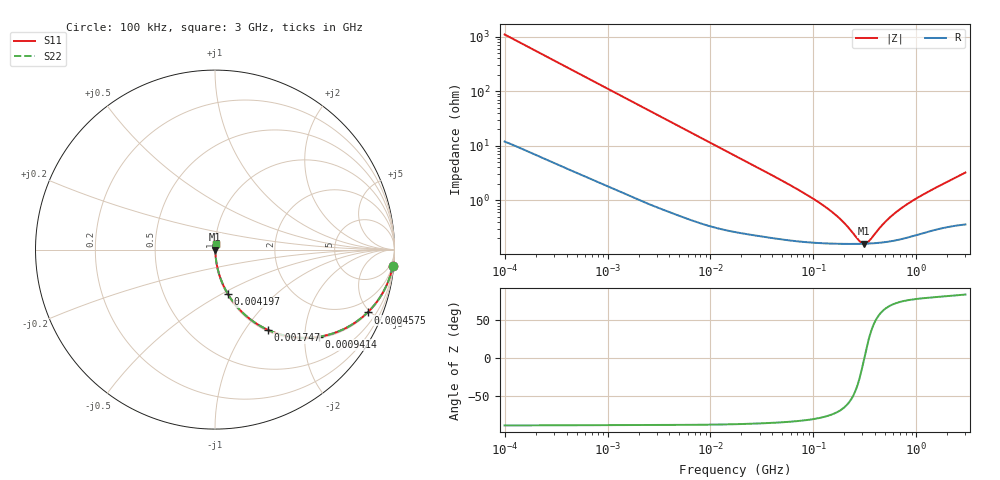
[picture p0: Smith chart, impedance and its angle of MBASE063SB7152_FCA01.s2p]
! MBASE063SB7152_FCA01  S-PARAMETER MODEL  ( Standard Model )
! Model Generated by TAIYO YUDEN Corporation (http://www.ty-top.com)
! Version 1.0
! TAIYO YUDEN Control No. 220601
! Copyright(c) 2020 TAIYO YUDEN CO.,LTD. All Rights Reserved.
! Product Description (link to TY-COMPAS)
! https://ds.yuden.co.jp/TYCOMPAS/or/detail?pn=MBASE063SB7152KFCA01&u=M
! Products Name : Multilayer Ceramic Capacitors
! Characteristics :
!  Capacitance : 1500 [pF] , Rated Voltage : 16 [V] , TCC : X7R
!  Case Size : 0.6 x 0.3 / 0.024 x 0.012 [mm/inch] , Thickness : 0.3 / 0.012 [mm/inch]
!  (Conditions: Temperature = 25 [degC] , DC Bias Voltage = 0 [V])
! External Node Assignments :
!  1  o---| |---o  2
! GND o---------o GND
! Frequency Range : 100kHz  -  3GHz  [ 401 STEP ]
# MHZ S RI R 50
! Freq[MHz].  S11 Real  S11 Imag  S21 Real  S21 Imag  S12 Real  S12 Imag  S22 Real  S22 Imag
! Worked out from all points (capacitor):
!   401 points, 100 kHz to 3 GHz, reference 50 ohm
!   read as one part in series: C = 1.46 nF near 105.3 kHz
!   lowest |Z| = 160 mohm at 310.6 MHz (marker M1)
!   series resonance near 313 MHz, so ESL is about 180 pH
!   S11 on the Smith chart (normalised r, x): 100 kHz: 1, -22; 457.5 kHz: 1.07, -4.83; 941.4 kHz: 1.04, -2.36; 1.747 MHz: 1.02, -1.28; 4.197 MHz: 1.01, -0.54; 3 GHz: 1.01, +0.06
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0.1  0.9907 -0.0907  0.00931 0.0907  0.00931 0.0907  0.9907 -0.0907
0.246461  0.9496 -0.2124  0.0504 0.2124  0.0504 0.2124  0.9496 -0.2124
0.457483  0.85 -0.35  0.15 0.35  0.15 0.35  0.85 -0.35
0.562235  0.7913 -0.3991  0.2087 0.3991  0.2087 0.3991  0.7913 -0.3991
0.941399  0.5812 -0.4854  0.4188 0.4854  0.4188 0.4854  0.5812 -0.4854
1.282589  0.4317 -0.4869  0.5683 0.4869  0.5683 0.4869  0.4317 -0.4869
1.747435  0.2941 -0.4468  0.7059 0.4468  0.7059 0.4468  0.2941 -0.4468
3.161081  0.1174 -0.312  0.8826 0.312  0.8826 0.312  0.1174 -0.312
4.197169  0.0721 -0.2481  0.9279 0.2481  0.9279 0.2481  0.0721 -0.2481
8.202936  0.0223 -0.1349  0.9777 0.1349  0.9777 0.1349  0.0223 -0.1349
17.7727  0.00666 -0.0636  0.9933 0.0636  0.9933 0.0636  0.00666 -0.0636
97.38194  0.00179 -0.0108  0.9982 0.0108  0.9982 0.0108  0.00179 -0.0108
167.3121  0.00162 -0.00499  0.9984 0.00499  0.9984 0.00499  0.00162 -0.00499
210.9903  0.00159 -0.00303  0.9984 0.00303  0.9984 0.00303  0.00159 -0.00303
280.1453  0.00159 -0.000832  0.9984 0.000832  0.9984 0.000832  0.00159 -0.000832
310.5665  0.0016 -5.72e-05  0.9984 5.72e-05  0.9984 5.72e-05  0.0016 -5.72e-05
353.2796  0.00161 0.000912  0.9984 -0.000912  0.9984 -0.000912  0.00161 0.000912
457.1373  0.00168 0.00291  0.9983 -0.00291  0.9983 -0.00291  0.00168 0.00291
547.5153  0.00177 0.00441  0.9982 -0.00441  0.9982 -0.00441  0.00177 0.00441
726.971  0.002 0.00702  0.998 -0.00702  0.998 -0.00702  0.002 0.00702
1016.304  0.00243 0.0107  0.9976 -0.0107  0.9976 -0.0107  0.00243 0.0107
3000  0.0046 0.0317  0.9954 -0.0317  0.9954 -0.0317  0.0046 0.0317
